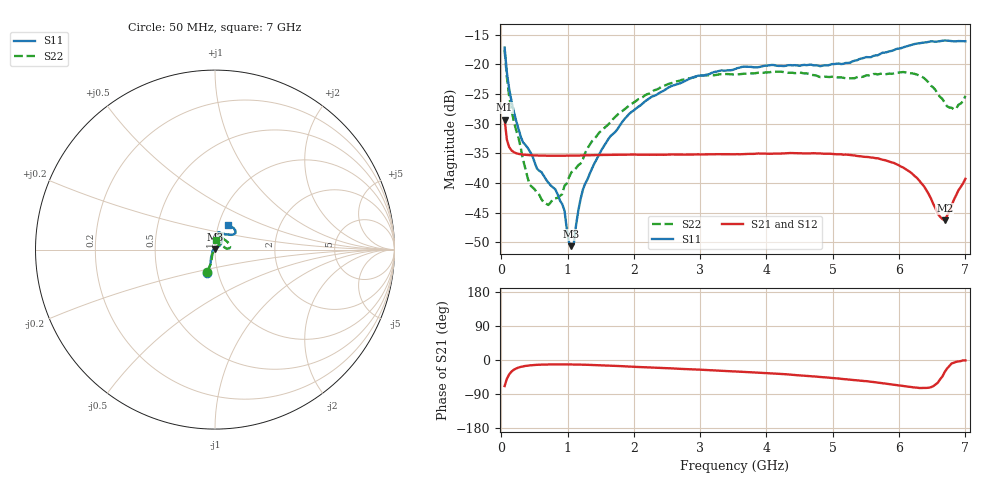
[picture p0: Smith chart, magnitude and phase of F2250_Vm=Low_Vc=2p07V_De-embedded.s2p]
! Integrated Device Technology
! Corporate Headquarters
! 6024 Silver Creek Valley Road
! San Jose, CA 95138  USA
! Phone:  1-408-284-8200
! Toll Free:  1-800-223-1366
! Webpage:  http://www.idt.com/
! Timing and RF Division
! 515 Groton Road, Suite 102
! Westford, MA 01886-6024
! Device:  F2250
! Description: Voltage Variable RF Attenuator
! Frequency:  50.0 -  6000.00 MHz
! Package:  3x3 mm Thin QFN Plastic Package: 16 pin
! Ports:  2 RF, 3 DC
!  Pin  1  = GND
!  Pin  2  = NC
!  Pin  3  = RF1  = Port 1
!  Pin  4  = NC
!  Pin  5  = GND
!  Pin  6  = GND
!  Pin  7  = GND
!  Pin  8  = GND
!  Pin  9  = NC
!  Pin 10  = RF2  = Port 2
!  Pin 11  = NC
!  Pin 12  = GND
!  Pin 13  = GND
!  Pin 14  = VCNTRL
!  Pin 15  = VDD
!  Pin 16  = VMODE
! Vcntrl:  2.070 Volts
! Vmode:  +0.000 Volts
! Vdd:  +3.30  Volts
! Current:  1.180 mA
! Data:  The device was measured on a the F2250 evaluation board which has
!  individual transmission lines to the RF pins.  Data was collected
!  using a calibrated network analyzer.  The evaluation board was
!  de-embedded using a TRL calibration technique.
!  The reference plane is the edge of the package pin.
! Misc:  SN 10
!  Action Tracker AT0258
! Date Measured:  2014-11-26
! Date:  2015-10-15  MJV
! Note:
!  Integrated Device Technology supplies this data as a sample of measured
!  data at the package pin for this product.  Your particular data for this
!  product may vary.
!  Data was taken at 25 degrees C.
!  Integrated Device Technology reserves the right to change this data at anytime.
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# GHz S dB R 50
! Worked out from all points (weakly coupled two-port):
!   201 points, 50 MHz to 7 GHz, reference 50 ohm
!   highest |S21| = -29.32 dB at 50 MHz (marker M1); lowest = -46.3 dB at 6.687 GHz (marker M2)
!   lowest |S11| = -50.7 dB at 1.058 GHz (marker M3), VSWR 1.01, Z = 49.8 + j0.246 ohm
!   |S11| at or under -10 dB: start of sweep to end of sweep
!   |S22| runs from -43.7 to -17.6 dB; largest |S21 - S12| = 6.5e-05
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0.05  -17.18 -108.6  -29.32 -68.8  -29.32 -68.8  -17.62 -109.4
0.08475  -21.44 -107.4  -32.75 -49.4  -32.75 -49.4  -22.23 -106.1
0.189  -28.00 -119.7  -34.82 -25.8  -34.82 -25.8  -29.63 -117.3
0.328  -33.16 -133.8  -35.24 -16.8  -35.24 -16.8  -36.09 -129.3
0.43225  -34.72 -144.5  -35.33 -14.1  -35.33 -14.1  -40.36 -156.1
0.71025  -39.96 -168.6  -35.42 -11.8  -35.42 -11.8  -43.72 141.3
0.91875  -43.57 158.0  -35.43 -11.6  -35.43 -11.6  -41.89 103.9
0.9535  -44.66 169.9  -35.43 -11.6  -35.43 -11.6  -40.48 105.2
1.023  -50.10 143.9  -35.42 -11.7  -35.42 -11.7  -39.01 86.4
1.05775  -50.67 122.7  -35.42 -11.8  -35.42 -11.8  -38.22 82.0
1.0925  -50.34 88.8  -35.40 -11.9  -35.40 -11.9  -37.91 77.2
1.162  -44.65 56.4  -35.39 -12.1  -35.39 -12.1  -37.01 66.8
1.2315  -41.11 43.9  -35.36 -12.3  -35.36 -12.3  -35.98 59.1
1.6485  -32.11 42.0  -35.28 -15.0  -35.28 -14.9  -29.73 51.5
2.37825  -24.88 47.3  -35.24 -20.7  -35.24 -20.7  -24.08 50.1
3.525  -20.80 72.5  -35.18 -30.1  -35.18 -30.2  -21.73 71.4
4.7065  -20.17 72.4  -34.99 -43.3  -35.00 -43.2  -21.83 70.4
5.85325  -17.82 40.5  -36.40 -63.8  -36.42 -63.8  -21.57 19.5
6.33975  -16.40 40.9  -40.11 -73.8  -40.13 -73.9  -22.07 5.3
6.68725  -15.99 48.8  -46.30 -32.0  -46.27 -31.8  -26.49 25.5
6.861  -16.13 55.1  -42.07 -4.9  -42.02 -4.9  -27.48 58.4
7  -16.12 63.2  -39.31 -1.0  -39.26 -1.1  -25.33 85.7
